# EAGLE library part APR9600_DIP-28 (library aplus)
SINGLE-CHIP VOICE RECORDING & PLAYBACK DEVICE FOR SINGLE 60 SECOND # Created by SCRIPT exported from Ultra Librarian Gold 5.3.88 Copyright © 1999-2010 # Tanvir Mohammed, Premier Farnell 2013-04-24 alf@cadsoft.de
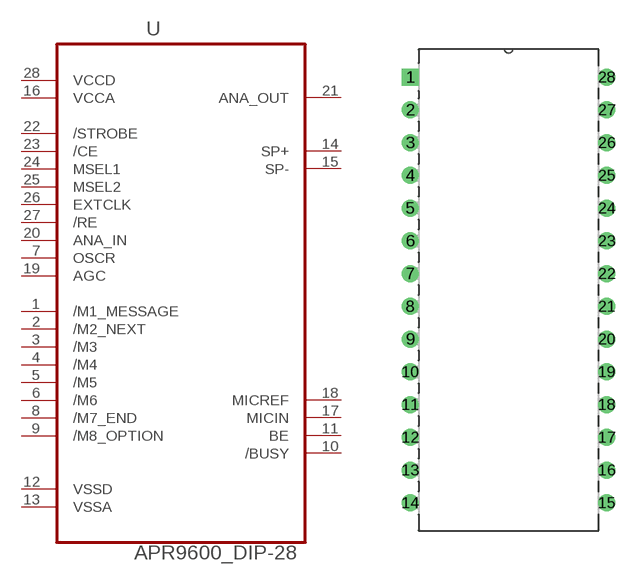
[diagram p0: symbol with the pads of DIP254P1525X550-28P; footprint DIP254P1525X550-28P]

Designator prefix U

## APR9600_DIP-28 (MPN: APR9600_DIP-28; OC_FARNELL: unknown; OC_NEWARK: unknown; PACKAGE: DIP-28; SUPPLIER: APLUS INTEGRATED CIRCUITS INC)  [DIP254P1525X550-28P]
1  /M1_MESSAGE  in
2  /M2_NEXT  in
3  /M3  in
4  /M4  in
5  /M5  in
6  /M6  in
7  OSCR  in
8  /M7_END  in
9  /M8_OPTION  in
10  /BUSY  in
11  BE  in
12  VSSD  pas
13  VSSA  pas
14  SP+  out
15  SP-  out
16  VCCA  pwr
17  MICIN  in
18  MICREF  in
19  AGC  in
20  ANA_IN  in
21  ANA_OUT  out
22  /STROBE  in
23  /CE  in
24  MSEL1  in
25  MSEL2  in
26  EXTCLK  in
27  /RE  in
28  VCCD  pwr

## Footprint DIP254P1525X550-28P (pad centres in mm)
# Created by Ultra Librarian Gold 5.3.88 Copyright © 1999-2010 # Tanvir Mohammed, Premier Farnell Origin corrected by alf@cadsoft.de
drill 0.813 pad 1.3 square: 1 -7.62,16.51
drill 0.813 pad 1.3: 2 -7.62,13.97; 3 -7.62,11.43; 4 -7.62,8.89; 5 -7.62,6.35; 6 -7.62,3.81; 7 -7.62,1.27; 8 -7.62,-1.27; 9 -7.62,-3.81; 10 -7.62,-6.35; 11 -7.62,-8.89; 12 -7.62,-11.43; 13 -7.62,-13.97; 14 -7.62,-16.51; 15 7.62,-16.51; 16 7.62,-13.97; 17 7.62,-11.43; 18 7.62,-8.89; 19 7.62,-6.35; 20 7.62,-3.81; 21 7.62,-1.27; 22 7.62,1.27; 23 7.62,3.81; 24 7.62,6.35; 25 7.62,8.89; 26 7.62,11.43; 27 7.62,13.97; 28 7.62,16.51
